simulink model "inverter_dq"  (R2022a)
settings: Solver=VariableStepAuto  StartTime=0.0  StopTime=T_sim  RelTol=1e-3
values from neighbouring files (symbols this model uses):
  grid_w = 2*pi*grid_freq    (= 1973.92088022)    [inverter_control_params_FR.m]
  I_step = 1    [inverter_control_params_FR.m]
  L = Lg+Lf    (= 0.00063)    [inverter_control_params_FR.m]
  R = Rf+Rg    (= 1)    [inverter_control_params_FR.m]
  T_step = 1e-4 * 1/grid_freq0    (= 2e-06)    [inverter_control_params_FR.m]
  Vgpk = 21.5    [inverter_control_params_FR.m]

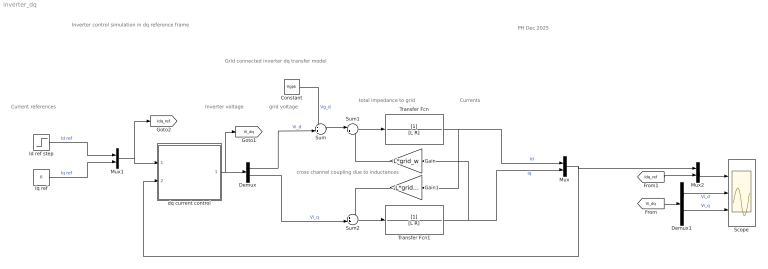
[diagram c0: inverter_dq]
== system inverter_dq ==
  note: grid voltage
  note: Grid connected inverter dq transfer model
  note: total impedance to grid
  note: cross channel coupling due to inductances
  note: Inverter control simulation in dq reference frame
  note: PH Dec 2025
  note: Currents
  note: Inverter voltage
  note: Current references
  Constant : Constant  Value=Vgpk
  Demux : Demux  Outputs=2
  Demux1 : Demux  Outputs=2
  Gain : Gain  Commented=on  Gain=L*grid_w
  Gain1 : Gain  Commented=on  Gain=-L*grid_w
  Id ref step : Step  Time=T_step  After=I_step  SampleTime=0
  Iq ref : Constant  Value=0
  Mux : Mux  Inputs=2
  Mux1 : Mux  Inputs=2
  Mux2 : Mux  Inputs=2
  Scope : Scope  NumInputPorts=3
  Sum : Sum  Inputs=-+|
  Sum1 : Sum  Inputs=|++
  Sum2 : Sum  Inputs=++|
  Transfer Fcn : TransferFcn  Denominator=[L R]
  Transfer Fcn1 : TransferFcn  Denominator=[L R]
  dq current control : Subsystem  ReferencedSubsystem=dq_current_control
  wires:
  dq current control/1 -> [Vi_dq], Demux/1
  Demux/1 -> Sum/2  "Vi_d"
  Mux/1 -> dq current control/2, Mux2/1
  Mux1/1 -> [Idq_ref], dq current control/1
  Sum/1 -> Sum1/1
  Demux/2 -> Sum2/2  "Vi_q"
  Transfer Fcn/1 -> Gain1/1, Mux/1  "Id"
  Transfer Fcn1/1 -> Gain/1, Mux/2  "Iq"
  Constant/1 -> Sum/1  "Vg_d"
  Iq ref/1 -> Mux1/2  "Iq ref"
  Id ref step/1 -> Mux1/1  "Id ref"
  Mux2/1 -> Scope/1
  [Idq_ref] -> Mux2/2
  [Vi_dq] -> Demux1/1
  Demux1/1 -> Scope/2  "Vi_d"
  Demux1/2 -> Scope/3  "Vi_q"
  Sum1/1 -> Transfer Fcn/1
  Gain/1 -> Sum1/2
  Gain1/1 -> Sum2/1
  Sum2/1 -> Transfer Fcn1/1
